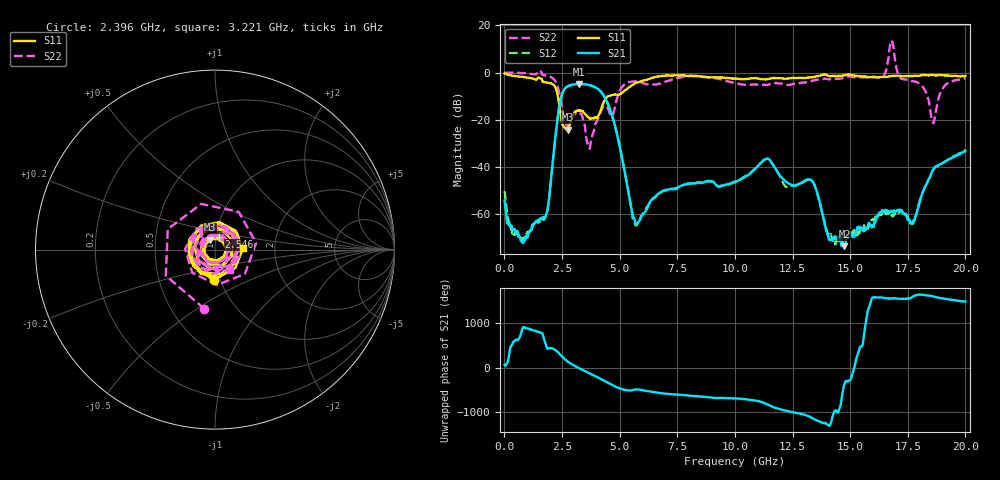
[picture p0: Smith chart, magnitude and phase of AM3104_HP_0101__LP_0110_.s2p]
!Created with skrf (http://scikit-rf.org).
# Hz S RI R 50.0
!freq ReS11 ImS11 ReS21 ImS21 ReS12 ImS12 ReS22 ImS22
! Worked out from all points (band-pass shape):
!   1601 points, 10 MHz to 20 GHz, reference 50 ohm
!   highest |S21| = -4.85 dB at 3.246 GHz (marker M1); lowest = -73.8 dB at 14.75 GHz (marker M2)
!   |S21| within 3 dB of the highest: 2.557 GHz to 4.161 GHz (1.603 GHz wide, 47.7 % of centre)
!   lowest |S11| = -24.3 dB at 2.746 GHz (marker M3), VSWR 1.13, Z = 47.1 + j5.19 ohm
!   |S11| at or under -10 dB: 2.32 GHz to 4.519 GHz (2.199 GHz wide, 64.3 % of centre)
!   |S22| runs from -32.3 to 13.6 dB; largest |S21 - S12| = 0.031
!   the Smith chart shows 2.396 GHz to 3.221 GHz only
!   S11 on the Smith chart (normalised r, x): 2.396 GHz: 0.93, -0.33; 2.546 GHz: 1.03, +0.15; 3.221 GHz: 1.37, +0.02
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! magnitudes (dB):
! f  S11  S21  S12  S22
! 10 MHz  -0.4  -54.3  -50.3  0.0
! 697.2 MHz  -1.8  -70.0  -70.3  -0.2
! 1.734 GHz  -4.0  -61.6  -62.4  -1.2
! 2.396 GHz  -15.3  -13.5  -13.5  -9.5
! 2.546 GHz  -22.6  -8.1  -8.1  -17.3
! 2.746 GHz  -24.3  -5.9  -5.9  -22.8
! 3.221 GHz  -16.2  -4.9  -5.0  -17.0
! 3.246 GHz  -16.3  -4.8  -4.9  -17.2
! 3.346 GHz  -16.3  -4.9  -5.0  -17.7
! 3.671 GHz  -19.1  -5.3  -5.4  -31.1
! 4.545 GHz  -9.9  -14.6  -14.7  -16.6
! 5.657 GHz  -4.6  -62.9  -64.1  -3.7
! 6.682 GHz  -1.6  -51.6  -51.6  -4.9
! 10.01 GHz  -2.7  -46.5  -46.7  -4.5
! 11.38 GHz  -2.9  -36.6  -36.8  -5.2
! 13.34 GHz  -2.1  -46.1  -46.0  -3.6
! 14.03 GHz  -1.3  -68.7  -68.6  -2.8
! 14.75 GHz  -1.2  -73.8  -69.6  -2.1
! 16.68 GHz  -1.6  -59.3  -60.1  7.2
! 17.7 GHz  -1.5  -63.6  -64.1  -3.7
! 18.6 GHz  -1.1  -41.3  -41.7  -21.4
! 20 GHz  -1.4  -33.3  -33.1  -2.5
